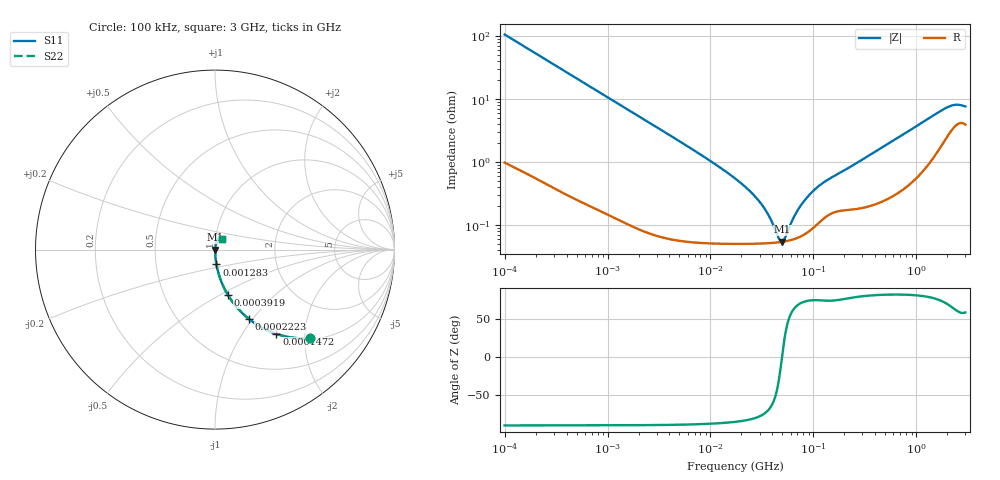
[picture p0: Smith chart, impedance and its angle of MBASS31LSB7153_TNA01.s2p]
! MBASS31LSB7153_TNA01  S-PARAMETER MODEL  ( Standard Model )
! Model Generated by TAIYO YUDEN Corporation (http://www.ty-top.com)
! Version 1.0
! TAIYO YUDEN Control No. 220601
! Copyright(c) 2013 TAIYO YUDEN CO.,LTD. All Rights Reserved.
! Product Description (link to TY-COMPAS)
! https://ds.yuden.co.jp/TYCOMPAS/or/detail?pn=MBASS31LSB7153KTNA01&u=M
! Products Name : Multilayer Ceramic Capacitors
! Characteristics :
!  Capacitance : 0.015 [uF] , Rated Voltage : 630 [V] , TCC : X7R
!  Case Size : 3.2 x 1.6 / 0.126 x 0.063 [mm/inch] , Thickness : 1.6 / 0.063 [mm/inch]
!  (Conditions: Temperature = 25 [degC] , DC Bias Voltage = 0 [V])
! External Node Assignments :
!  1  o---| |---o  2
! GND o---------o GND
! Frequency Range : 100kHz  -  3GHz  [ 401 STEP ]
# MHZ S RI R 50
! Freq[MHz].  S11 Real  S11 Imag  S21 Real  S21 Imag  S12 Real  S12 Imag  S22 Real  S22 Imag
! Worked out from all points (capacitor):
!   401 points, 100 kHz to 3 GHz, reference 50 ohm
!   read as one part in series: C = 15 nF near 105.3 kHz
!   lowest |Z| = 54.2 mohm at 49.83 MHz (marker M1)
!   series resonance near 49.54 MHz, so ESL is about 690 pH
!   S11 on the Smith chart (normalised r, x): 100 kHz: 1.02, -2.11; 147.2 kHz: 1.01, -1.44; 222.3 kHz: 1.01, -0.96; 391.9 kHz: 1.01, -0.54; 1.283 MHz: 1.00, -0.17; 3 GHz: 1.08, +0.13
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0.1  0.5272 -0.4946  0.4728 0.4946  0.4728 0.4946  0.5272 -0.4946
0.147195  0.3425 -0.4696  0.6575 0.4696  0.6575 0.4696  0.3425 -0.4696
0.222319  0.1882 -0.3857  0.8118 0.3857  0.8118 0.3857  0.1882 -0.3857
0.391939  0.0713 -0.2517  0.9287 0.2517  0.9287 0.2517  0.0713 -0.2517
0.562235  0.0369 -0.1825  0.9631 0.1825  0.9631 0.1825  0.0369 -0.1825
1.282589  0.00814 -0.0829  0.9919 0.0829  0.9919 0.0829  0.00814 -0.0829
3.161081  0.00181 -0.0339  0.9982 0.0339  0.9982 0.0339  0.00181 -0.0339
17.7727  0.00053 -0.0053  0.9995 0.0053  0.9995 0.0053  0.00053 -0.0053
24.84619  0.000514 -0.00326  0.9995 0.00326  0.9995 0.00326  0.000514 -0.00326
31.3325  0.000513 -0.00208  0.9995 0.00208  0.9995 0.00208  0.000513 -0.00208
37.52708  0.000518 -0.00123  0.9995 0.00123  0.9995 0.00123  0.000518 -0.00123
46.11977  0.000533 -0.000315  0.9995 0.000315  0.9995 0.000315  0.000533 -0.000315
49.82709  0.000542 2.59e-05  0.9995 -2.59e-05  0.9995 -2.59e-05  0.000542 2.59e-05
52.46276  0.000549 0.000254  0.9995 -0.000254  0.9995 -0.000254  0.000549 0.000254
62.83488  0.000588 0.00107  0.9994 -0.00107  0.9994 -0.00107  0.000588 0.00107
71.47675  0.000635 0.00167  0.9994 -0.00167  0.9994 -0.00167  0.000635 0.00167
97.38194  0.000881 0.00323  0.9991 -0.00323  0.9991 -0.00323  0.000881 0.00323
132.6759  0.00137 0.00484  0.9986 -0.00484  0.9986 -0.00484  0.00137 0.00484
547.5153  0.00306 0.0198  0.9969 -0.0198  0.9969 -0.0198  0.00306 0.0198
1935.725  0.027 0.0647  0.973 -0.0647  0.973 -0.0647  0.027 0.0647
2378.954  0.0403 0.0666  0.9597 -0.0666  0.9597 -0.0666  0.0403 0.0666
3000  0.0416 0.0602  0.9584 -0.0602  0.9584 -0.0602  0.0416 0.0602
